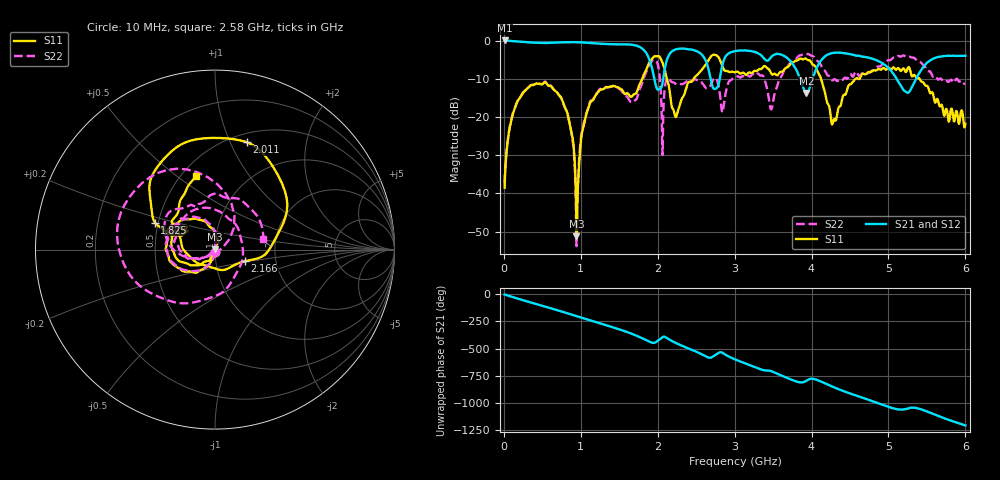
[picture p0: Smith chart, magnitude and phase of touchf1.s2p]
!  15/09/2025  16:03:41
! Ref Plane: 0.000 mm
# MHZ S MA R  50
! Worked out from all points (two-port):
!   1001 points, 10 MHz to 6 GHz, reference 50 ohm
!   highest |S21| = 0.02 dB at 10 MHz (marker M1); lowest = -13.7 dB at 3.933 GHz (marker M2)
!   |S21| within 3 dB of the highest: start of sweep to 1.841 GHz; 2.177 GHz to 2.527 GHz (350.2 MHz wide, 14.9 % of centre)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
!   lowest |S11| = -51.3 dB at 944.4 MHz (marker M3), VSWR 1.01, Z = 50.1 + j0.268 ohm
!   |S11| at or under -10 dB: start of sweep to 1.8 GHz; 4.124 GHz to 4.573 GHz (449.9 MHz wide, 10.3 % of centre); 5.403 GHz to end of sweep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
!   |S22| runs from -53.8 to -3.5 dB; largest |S21 - S12| = 0.012
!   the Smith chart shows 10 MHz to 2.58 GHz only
!   S11 on the Smith chart (normalised r, x): 10 MHz: 1.00, -0.02; 1.825 GHz: 0.48, +0.17; 2.011 GHz: 0.59, +1.15; 2.166 GHz: 1.38, -0.18; 2.58 GHz: 0.59, +0.59
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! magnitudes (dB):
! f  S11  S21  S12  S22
! 10 MHz  -38.5  0.0  0.0  -37.2
! 165.7 MHz  -16.5  -0.2  -0.3  -16.4
! 537.1 MHz  -10.9  -0.7  -0.7  -10.7
! 824.6 MHz  -18.9  -0.4  -0.5  -19.2
! 944.4 MHz  -51.3  -0.4  -0.5  -53.8
! 1.01 GHz  -24.9  -0.5  -0.5  -24.3
! 1.232 GHz  -13.4  -0.8  -0.9  -13.1
! 1.825 GHz  -8.7  -2.6  -2.6  -9.5
! 2.011 GHz  -4.1  -12.8  -12.9  -7.1
! 2.065 GHz  -5.9  -11.0  -11.1  -29.9
! 2.166 GHz  -15.0  -3.2  -3.3  -10.6
! 2.58 GHz  -7.5  -3.8  -3.9  -11.2
! 2.747 GHz  -3.8  -12.7  -12.7  -9.7
! 2.843 GHz  -6.8  -6.2  -6.2  -18.8
! 3.005 GHz  -8.3  -2.8  -2.8  -9.9
! 3.478 GHz  -8.7  -4.2  -4.2  -18.0
! 3.933 GHz  -4.9  -13.7  -13.7  -3.5
! 4.005 GHz  -6.0  -10.4  -10.4  -4.0
! 4.287 GHz  -20.8  -3.2  -3.3  -10.2
! 5.006 GHz  -7.1  -7.4  -7.4  -5.1
! 5.251 GHz  -7.2  -13.7  -13.7  -4.1
! 6 GHz  -21.8  -4.0  -4.0  -11.3
